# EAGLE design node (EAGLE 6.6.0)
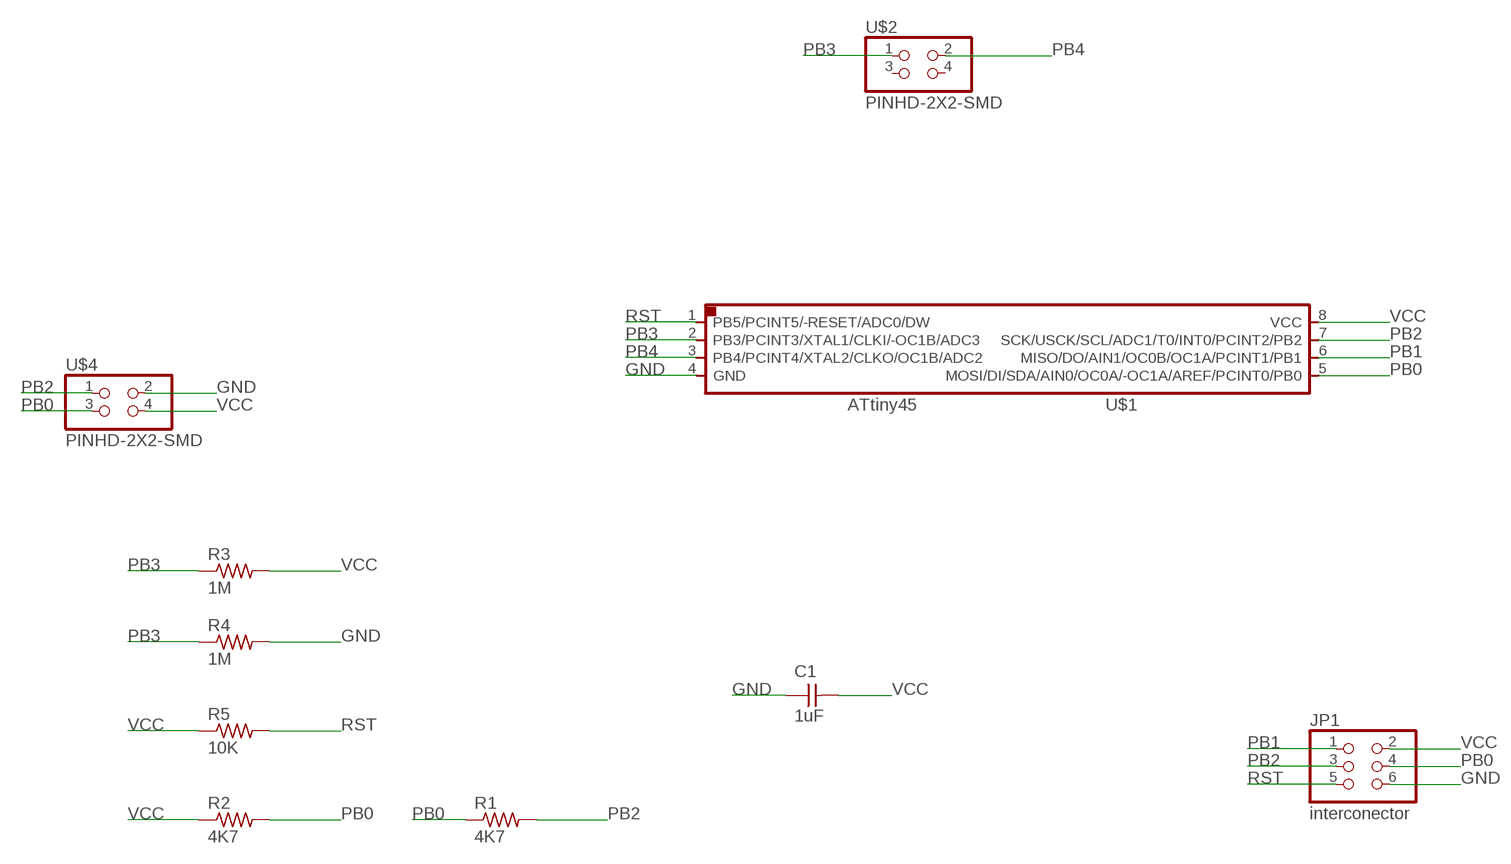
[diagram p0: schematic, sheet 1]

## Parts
C1  1uF  CAP-UNPOLARIZED  [C1206]
JP1  interconector  PINHD-2X3-SMD  [2X03SMD]
R1  4K7  RES-US1206FAB  [R1206FAB]
R2  4K7  RES-US1206FAB  [R1206FAB]
R3  1M  RES-US1206FAB  [R1206FAB]
R4  1M  RES-US1206FAB  [R1206FAB]
R5  10K  RES-US1206FAB  [R1206FAB]
U$1  ATTINY45SI  [SOIC8]
U$2  PINHD-2X2-SMD  [2X02SMD]
U$4  PINHD-2X2-SMD  [2X02SMD]

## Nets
GND [ground]: C1.1 JP1.6 R4.2 U$1.4(GND) U$4.2
PB0: JP1.4 R1.1 R2.2 U$1.5(MOSI/DI/SDA/AIN0/OC0A/-OC1A/AREF/PCINT0/PB0) U$4.3
PB1: JP1.1 U$1.6(MISO/DO/AIN1/OC0B/OC1A/PCINT1/PB1)
PB2: JP1.3 R1.2 U$1.7(SCK/USCK/SCL/ADC1/T0/INT0/PCINT2/PB2) U$4.1
PB3: R3.1 R4.1 U$1.2(PB3/PCINT3/XTAL1/CLKI/-OC1B/ADC3) U$2.1
PB4: U$1.3(PB4/PCINT4/XTAL2/CLKO/OC1B/ADC2) U$2.2
RST: JP1.5 R5.2 U$1.1(PB5/PCINT5/-RESET/ADC0/DW)
VCC: C1.2 JP1.2 R2.1 R3.2 R5.1 U$1.8(VCC) U$4.4
Unconnected: U$2.3 U$2.4

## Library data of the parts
C1 = fab:CAP-UNPOLARIZED
JP1 = fab:PINHD-2X3-SMD: PIN HEADER
R1-R5 = fab:RES-US: Resistor (US Symbol)
U$1 = fab:ATTINY45
U$2 U$4 = fab:PINHD-2X2-SMD

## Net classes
0 default: width 0.406 mm, drill 0.406 mm, clearance 0.406 mm
1 ground: width 0.406 mm, drill 0.406 mm, clearance 0.406 mm

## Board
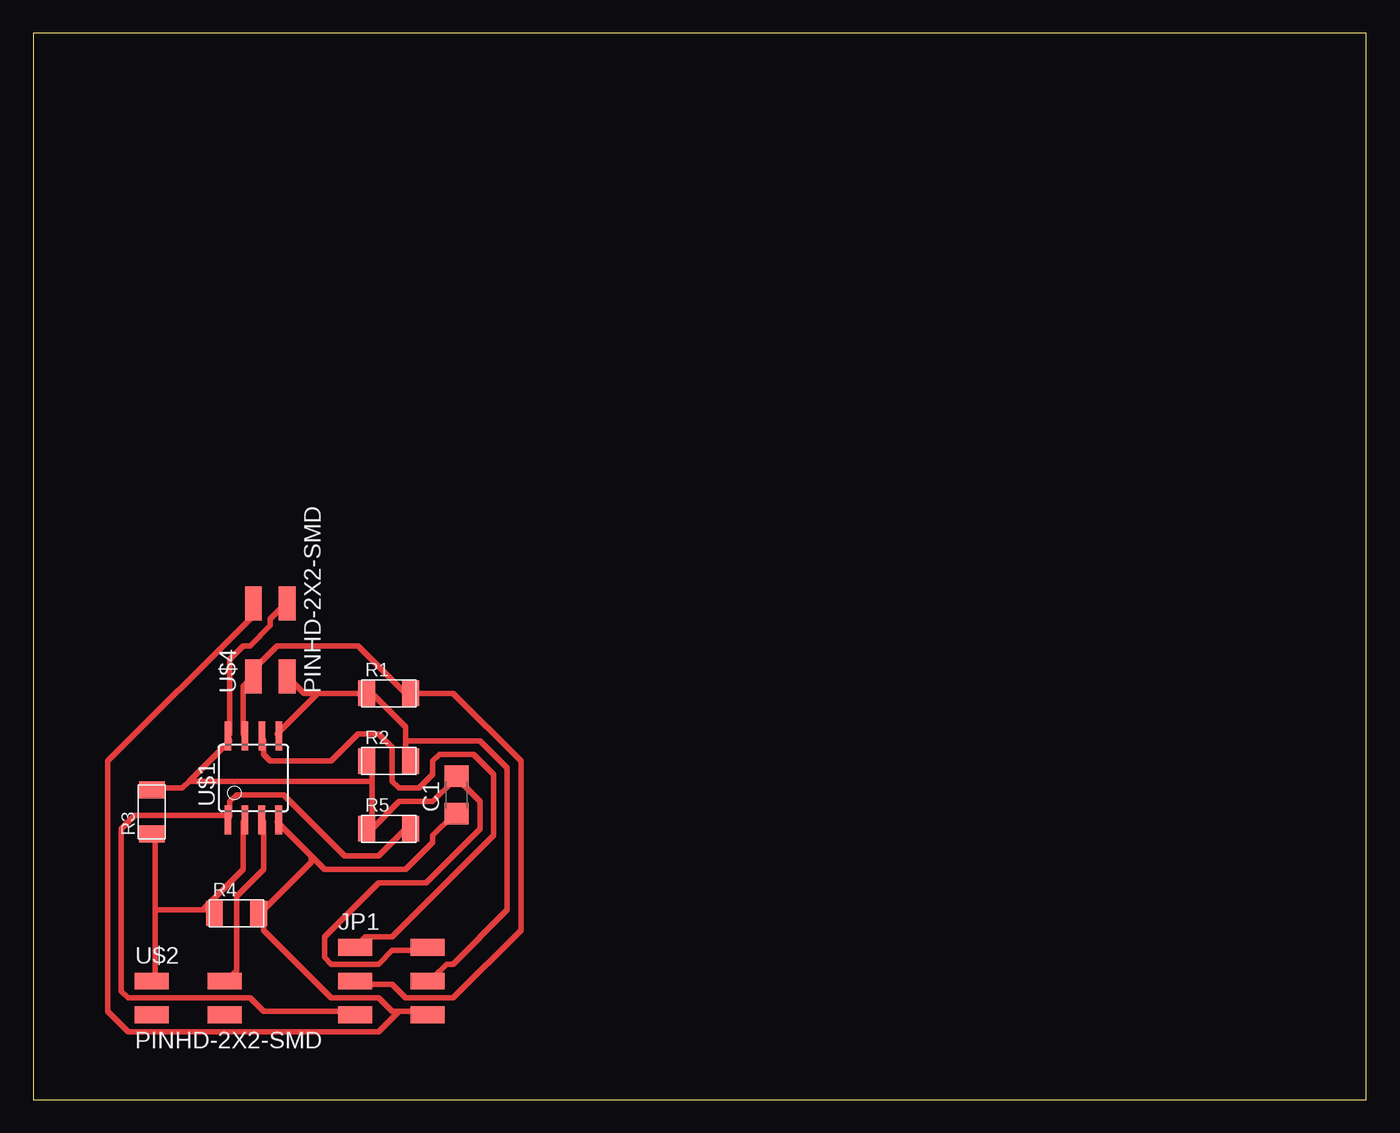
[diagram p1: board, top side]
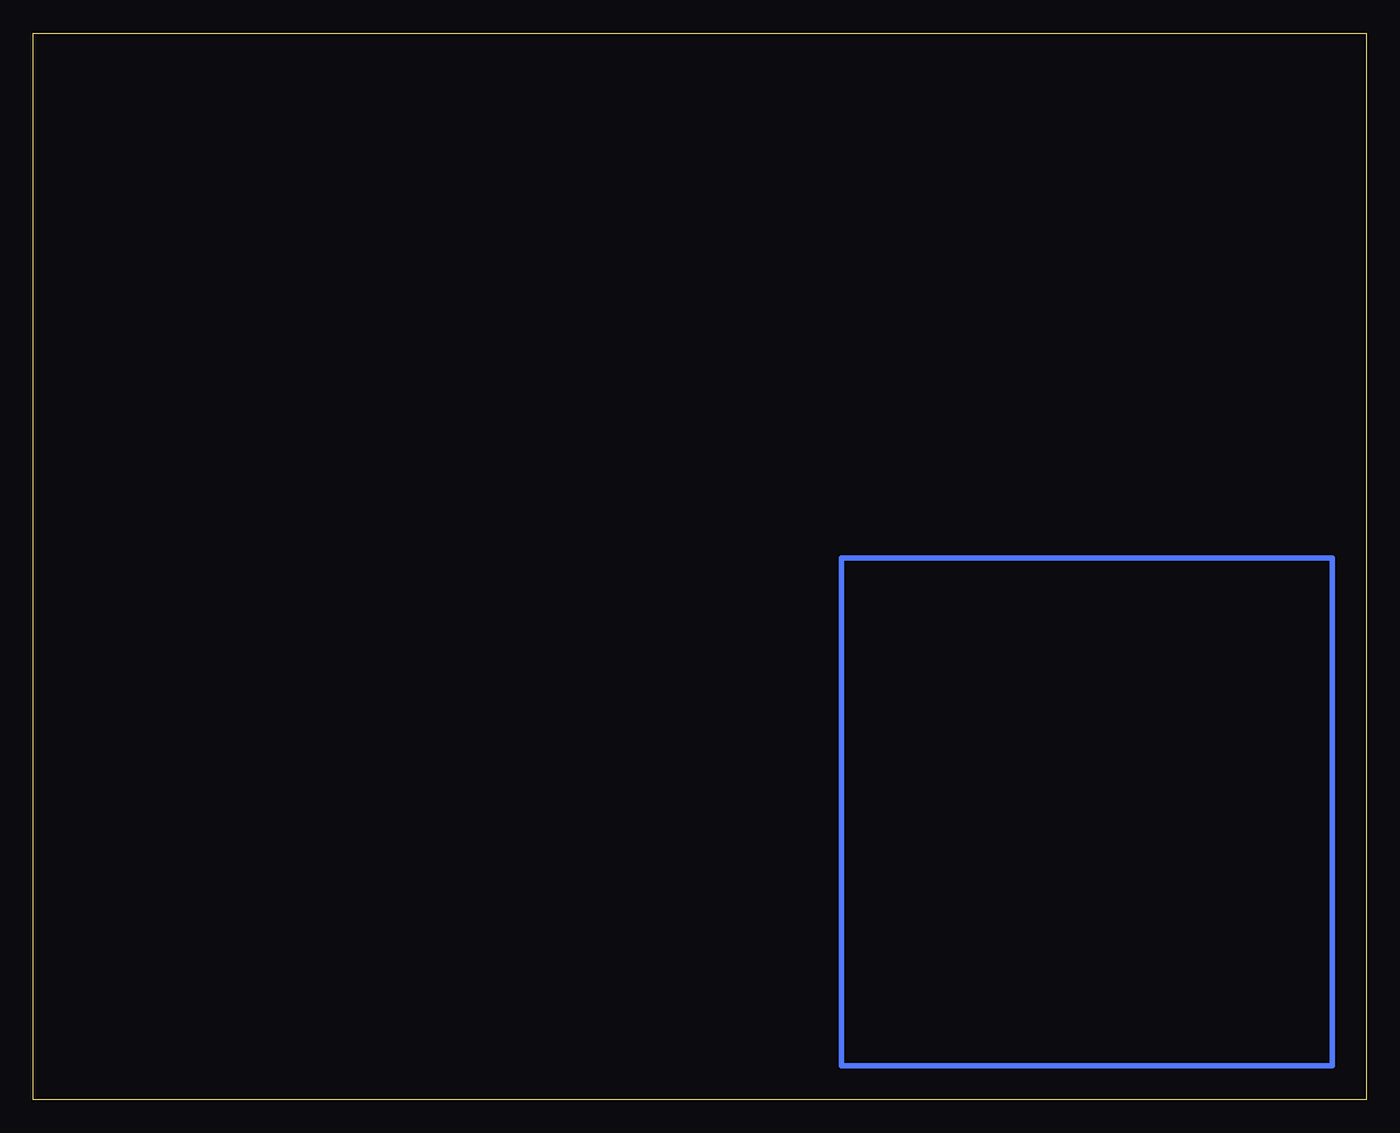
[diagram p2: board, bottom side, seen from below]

Size 100 x 80 mm. Coordinates in mm from the lower left corner, seen from the top.
Outline: 0,0 100,0 100,80 0,80 0,0
Copper layers (1*16): Top 0.035mm / dielectric 1.5mm / Bottom 0.035mm
Design rules "default *": minimum track width 10mil, minimum drill 24mil, track to track 16mil, track to pad 16mil, pad to pad 16mil, via to via 16mil, smd to smd 16mil, copper to edge 40mil, drill to drill 8mil, minimum pad ring 10mil, minimum via ring 8mil, stop-mask expansion 4mil, vias tented up to drill 0mil, thermal gap 10mil

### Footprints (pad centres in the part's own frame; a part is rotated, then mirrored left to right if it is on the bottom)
C1206 = smd 1.6 x 1.8: 1 -1.4,0; 2 1.4,0
2X03SMD = smd 2.54 x 1.27: 1 -2.54,2.54; 2 2.92,2.54; 3 -2.54,0; 4 2.92,0; 5 -2.54,-2.54; 6 2.92,-2.54
R1206FAB = smd 1.27 x 1.905: 1 -1.651,0; 2 1.651,0
SOIC8 = smd 0.5 x 2.2: 1 -1.905,-3.154; 2 -0.645,-3.154; 3 0.625,-3.154; 4 1.895,-3.154; 5 1.905,3.154; 6 0.635,3.154; 7 -0.635,3.154; 8 -1.905,3.154
2X02SMD = smd 2.54 x 1.27: 1 -2.54,1.27; 2 2.92,1.27; 3 -2.54,-1.27; 4 2.92,-1.27

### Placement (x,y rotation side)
C1  31.75,22.86 90 top
JP1  26.67,8.89 0 top
R1  26.67,30.48 0 top
R2  26.67,25.4 0 top
R3  8.89,21.59 90 top
R4  15.24,13.97 0 top
R5  26.67,20.32 0 top
U$1  16.51,24.13 0 top
U$2  11.43,7.62 0 top
U$4  17.78,34.29 90 top

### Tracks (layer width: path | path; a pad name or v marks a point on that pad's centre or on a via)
GND
  Top 0.406: 20.83,18.29 18.29,20.83 U$1.4 | 20.83,18.29 21.84,17.27 27.94,17.27 29.97,19.3 29.97,19.81 31.5,21.34 C1.1 | 20.83,18.29 20.83,17.78 17.27,14.22 R4.2 17.27,13.72 17.27,12.7 22.35,7.62 25.91,7.62 26.92,6.6 27.43,6.6 | 27.43,6.6 29.46,6.6 JP1.6 | 27.43,6.6 25.91,5.08 7.11,5.08 5.59,6.6 5.59,25.4 16.26,36.07 16.26,37.08 U$4.2
N$1
  Bottom 0.406: 2.54,2.54 2.54,40.64 39.37,40.64 39.37,2.54 2.54,2.54
PB0
  Top 0.406: 21.34,30.48 20.32,30.48 U$4.3 | 21.34,30.48 R1.1 25.4,30.48 27.94,27.94 27.94,26.92 | 27.94,26.92 27.94,25.4 R2.2 | 21.34,30.48 18.29,27.43 U$1.5 | 27.94,26.92 33.53,26.92 35.56,24.89 35.56,14.22 31.5,10.16 30.99,10.16 29.97,9.14 JP1.4
PB1
  Top 0.406: JP1.1 24.89,12.19 26.92,12.19 34.54,19.81 34.54,24.38 33.02,25.91 30.48,25.91 29.97,25.4 29.97,24.38 28.96,23.37 27.43,23.37 26.92,23.88 26.92,26.42 25.91,27.43 24.38,27.43 22.35,25.4 17.78,25.4 17.27,25.91 17.27,26.92 U$1.6
PB2
  Top 0.406: U$1.7 15.75,27.43 15.75,30.99 U$4.1 16.26,32 18.29,34.04 24.38,34.04 27.94,30.48 R1.2 31.5,30.48 36.58,25.4 36.58,12.7 31.5,7.62 27.94,7.62 26.92,8.64 24.38,8.64 JP1.3
PB3
  Top 0.406: 9.14,14.22 9.14,9.14 U$2.1 | 9.14,14.22 9.14,19.81 R3.1 | 9.14,14.22 12.7,14.22 | 12.7,14.22 13.21,14.22 R4.1 | 12.7,14.22 15.75,17.27 15.75,20.83 U$1.2
PB4
  Top 0.406: U$1.3 17.27,20.83 17.27,17.27 15.24,15.24 15.24,9.65 14.73,9.14 U$2.2
RST
  Top 0.406: 14.73,21.34 14.73,22.35 15.24,22.86 18.8,22.86 23.37,18.29 25.91,18.29 27.94,20.32 R5.2 | 14.73,21.34 7.62,21.34 6.6,20.32 6.6,8.13 7.11,7.62 16.26,7.62 17.27,6.6 23.88,6.6 JP1.5 | 14.73,21.34 U$1.1
VCC
  Top 0.406: 25.4,20.32 27.43,22.35 29.97,22.35 31.5,23.88 C1.2 32,23.88 33.53,22.35 33.53,20.32 29.46,16.26 25.91,16.26 21.84,12.19 21.84,10.67 22.35,10.16 25.91,10.16 26.92,11.18 29.46,11.18 JP1.2 | 25.4,20.32 25.4,23.88 | 25.4,23.88 25.4,25.4 R2.1 | 25.4,20.32 R5.1 | 11.68,23.88 14.73,26.92 U$1.8 14.73,27.43 14.73,33.02 15.75,34.04 16.26,34.04 17.78,35.56 17.78,36.07 18.8,37.08 U$4.4 | 11.68,23.88 11.18,23.37 9.14,23.37 R3.2 | 11.68,23.88 25.4,23.88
